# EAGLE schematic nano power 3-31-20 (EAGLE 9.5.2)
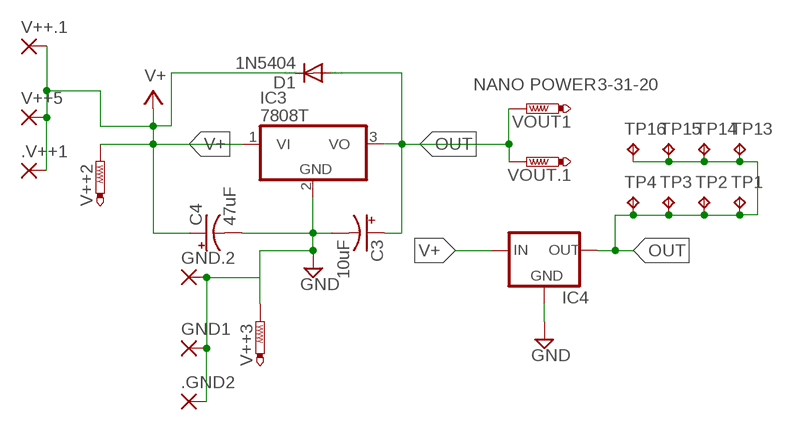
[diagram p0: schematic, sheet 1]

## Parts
.GND2  2,54/1,0  [2,54/1,0]
.V++1  2,54/1,0  [2,54/1,0]
C3  10uF  CPOL-USE3.5-10  [E3,5-10]
C4  47uF  CPOL-USE3.5-10  [E3,5-10]
D1  1N5404  1N4148DO35-10  [DO35-10]
GND1  2,54/1,0  [2,54/1,0]
GND.2  2,54/1,0  [2,54/1,0]
IC3  7808T  7805T  [TO220H]
IC4  78LXX  [78LXX]
TP1  TPPAD1-13  [P1-13]
TP2  TPPAD1-13  [P1-13]
TP3  TPPAD1-13  [P1-13]
TP4  TPPAD1-13  [P1-13]
TP13  TPPAD1-13  [P1-13]
TP14  TPPAD1-13  [P1-13]
TP15  TPPAD1-13  [P1-13]
TP16  TPPAD1-13  [P1-13]
V++2  PTR1PAD1-13Y  [P1-13Y]
V++3  PTR1PAD1-13Y  [P1-13Y]
V++5  2,54/1,0  [2,54/1,0]
V++.1  2,54/1,0  [2,54/1,0]
VOUT1  PTR1PAD1-13Y  [P1-13Y]
VOUT.1  PTR1PAD1-13Y  [P1-13Y]

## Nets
GND: .GND2.1(P) C3.- C4.- GND1.1(P) GND.2.1(P) IC3.2(GND) IC4.GND V++3.TP
OUT: C3.+ D1.A IC3.3(VO) IC4.OUT TP1.TP TP2.TP TP3.TP TP4.TP TP13.TP TP14.TP TP15.TP TP16.TP VOUT1.TP VOUT.1.TP
V+: .V++1.1(P) C4.+ D1.C IC3.1(VI) IC4.IN V++2.TP V++5.1(P) V++.1.1(P)

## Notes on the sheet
- NANO POWER | 3-31-20

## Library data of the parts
.GND2 .V++1 GND1 GND.2 V++5 V++.1 = wirepad-NONAMES:2,54/1,0: THROUGH-HOLE PAD
C3 C4 = rcl:CPOL-US: POLARIZED CAPACITOR, American symbol; SPICEPREFIX: C
D1 = diode:1N4148: DIODE
IC3 = linear:78*: Positive VOLTAGE REGULATOR Source: http://cache.national.com/ds/LM/LM78L05.pdf http://www.fairchildsemi.com/ds/LM/LM7805.pdf
IC4 = v-reg:78LXX: VOLTAGE REGULATOR
TP1-TP4 TP13-TP16 = testpad-CL:TP: Test pad NO NAME
V++2 V++3 VOUT1 VOUT.1 = testpad-CL:PTR1: TEST PIN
